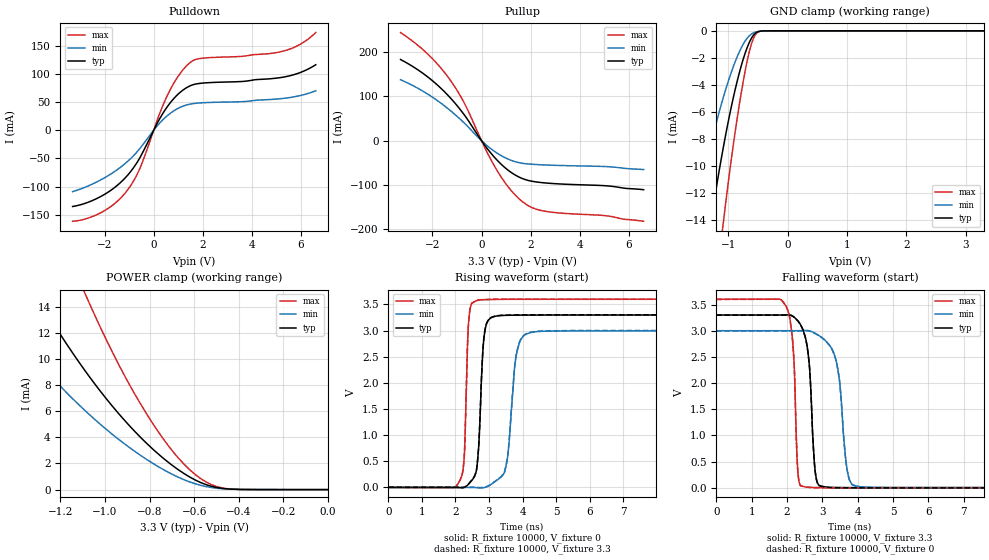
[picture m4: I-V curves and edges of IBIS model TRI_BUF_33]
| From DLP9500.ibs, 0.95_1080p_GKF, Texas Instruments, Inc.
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[Model]   TRI_BUF_33
Model_type  3-state
Enable   Active-High
Vref =   0
Rref =   10000
Cref =   0p
Vmeas =   1.5
| variable   typ   min   max
C_comp   1.64pF   1.51pF   2.01pF
| C_pullup   3.64pF   2.66pF   4.74pF
| C_pulldown   2.77pF   1.94pF   3.37pF
| C_tri-state   1.64pF   1.51pF   2.01pF
[Temperature Range]   40   125   -40
| Ambient temperature   25   110   -40
[Voltage range]   3.3   3   3.6
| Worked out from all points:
|   slope of the pulldown table from 0 to 0.495 V, typ, clamps not added: 12.9 ohm
|   slope of the pullup table from 0 to 0.495 V, typ, clamps not added: 13.9 ohm
|   GND clamp passes 1 mA (typ) near -0.66 V on its own axis
|   POWER clamp passes 1 mA (typ) near -0.62 V on its own axis
|   rising waveform, R_fixture 10000, V_fixture 0: 20-80 % time 141ps typ, 224ps min, 96.6ps max; typ from 0 V to 3.3 V
|   falling waveform, R_fixture 10000, V_fixture 3.3: 20-80 % time 174ps typ, 253ps min, 128ps max; typ from 3.3 V to 0.004 V
|   rising waveform, R_fixture 10000, V_fixture 3.3: 20-80 % time 141ps typ, 224ps min, 96.6ps max; typ from 0.004 V to 3.3 V
|   falling waveform, R_fixture 10000, V_fixture 0: 20-80 % time 174ps typ, 253ps min, 127ps max; typ from 3.3 V to 0 V
[GND Clamp]
| TRI_BUF_33
|   Voltage   I(typ)   I(min)   I(max)
-3.3V     -90.74mA   -64.34mA   -120.4mA
-1.58V    -23.02mA   -14.24mA   -35.11mA
-1.315V   -14.82mA   -8.851mA   -23.44mA
-1.28V    -13.82mA   -8.21mA    -21.98mA
-1.08V    -8.591mA   -4.902mA   -14.14mA
-935mV    -5.377mA   -2.918mA   -9.123mA
-795mV    -2.828mA   -1.398mA   -4.995mA
-670mV    -1.125mA   -492uA     -2.021mA
-575mV    -328.8uA   -155.1uA   -571.2uA
-500mV    -70.88uA   -51.22uA   -102.5uA
-375mV    -2.475uA   -4.552uA   -1.459uA
3.3V      49.59pA    1.106uA    33.03pA
[POWER Clamp]
| TRI_BUF_33
|   Voltage   I(typ)   I(min)   I(max)
-3.3V     108mA      77.88mA    156.4mA
-1.545V   22.36mA    15.03mA    36.12mA
-1.3V     14.64mA    9.77mA     23.97mA
-1.095V   9.233mA    6.138mA    15.22mA
-1.075V   8.762mA    5.822mA    14.45mA
-945mV    5.943mA    3.931mA    9.788mA
-805mV    3.41mA     2.22mA     5.575mA
-705mV    1.945mA    1.23mA     3.121mA
-595mV    732.7uA    446uA      1.151mA
-525mV    266uA      165.6uA    400.3uA
-440mV    41.44uA    31.47uA    49.29uA
-48.03fV  49.59pA    201.8pA    43.32pA
[Pulldown]
| TRI_BUF_33
|   Voltage   I(typ)   I(min)   I(max)
-3.3V     -135.4mA   -109mA     -161.7mA
-2.03V    -114.7mA   -85.13mA   -143.6mA
-1.045V   -78.98mA   -54.56mA   -105mA
-555mV    -48.27mA   -31.88mA   -67.09mA
220mV     18.6mA     11.64mA    27.17mA
600mV     44.67mA    27.61mA    65.86mA
1.045V    66.29mA    40.16mA    99.13mA
1.5V      79.42mA    46.79mA    121mA
1.97V     83.91mA    48.95mA    128.2mA
5.21V     94.09mA    56.42mA    140.1mA
5.945V    102.4mA    61.6mA     152.4mA
6.6V      116.6mA    70.3mA     173.8mA
[Pullup]
| TRI_BUF_33
|   Voltage   I(typ)   I(min)   I(max)
-3.3V     183.6mA    137.8mA    244.4mA
-2.205V   144.7mA    105.8mA    196.6mA
-1.31V    99.19mA    69.94mA    139.7mA
-695mV    57.8mA     39.52mA    84.19mA
140mV     -10.9mA    -7.086mA   -16.47mA
615mV     -42.85mA   -27.33mA   -65.74mA
1.15V     -69.42mA   -43.04mA   -108.8mA
1.68V     -85.76mA   -51.11mA   -138.3mA
2.105V    -91.99mA   -53.34mA   -152.2mA
2.63V     -95.51mA   -54.82mA   -159.7mA
5.005V    -101.5mA   -58.24mA   -169.1mA
6.6V      -110.6mA   -65.14mA   -182mA
[Ramp]
| TRI_BUF_33
| variable   typ   min   max
dV/dt_r   1.98/1.49E-10   1.80/2.36E-10   2.16/1.03E-10
dV/dt_f   1.98/1.77E-10   1.80/2.56E-10   2.16/1.29E-10
R_load = 10000
[Rising Waveform]
| TRI_BUF_33
R_fixture =   10000
C_fixture =   0
L_fixture =   0
V_fixture =   0
V_fixture_min = 0
V_fixture_max = 0
|   Time   V(typ)   V(min)   V(max)
0s        920.7pV    4.06nV     601pV
2.14ns    -4.487mV   139.3uV    142.8mV
2.265ns   1.174mV    246.3uV    626.8mV
2.4ns     71.01mV    -37.67uV   3.22V
2.665ns   557.9mV    -4.992mV   3.577V
2.93ns    3.137V     11.71mV    3.591V
3.47ns    3.289V     311.6mV    3.596V
3.815ns   3.293V     2.54V      3.597V
4.225ns   3.295V     2.959V     3.597V
23ns      3.296V     2.994V     3.597V
[Falling Waveform]
| TRI_BUF_33
R_fixture =   10000
C_fixture =   0
L_fixture =   0
V_fixture =   3.3
V_fixture_min = 3
V_fixture_max = 3.6
|   Time   V(typ)   V(min)   V(max)
0s        3.3V       3V         3.6V
1.985ns   3.302V     3V         3.457V
2.18ns    3.271V     3V         2.632V
2.32ns    3.18V      3V         232.1mV
2.5ns     2.923V     3.004V     19.74mV
2.8ns     313.1mV    2.951V     6.608mV
2.98ns    31.35mV    2.876V     4.673mV
3.395ns   6.65mV     2.423V     3.14mV
3.95ns    4.082mV    37.68mV    2.783mV
23ns      3.639mV    5.256mV    2.73mV
[Rising Waveform]
| TRI_BUF_33
R_fixture =   10000
C_fixture =   0
L_fixture =   0
V_fixture =   3.3
V_fixture_min = 3
V_fixture_max = 3.6
|   Time   V(typ)   V(min)   V(max)
0s        3.639mV    5.256mV    2.73mV
2.14ns    -827.2uV   5.394mV    146.2mV
2.265ns   4.91mV     5.498mV    634mV
2.4ns     75.12mV    5.212mV    3.226V
2.665ns   569mV      298.7uV    3.58V
2.93ns    3.143V     17.28mV    3.594V
3.47ns    3.293V     324.1mV    3.599V
3.815ns   3.297V     2.556V     3.6V
4.225ns   3.299V     2.966V     3.6V
23ns      3.3V       3V         3.6V
[Falling Waveform]
| TRI_BUF_33
R_fixture =   10000
C_fixture =   0
L_fixture =   0
V_fixture =   0
V_fixture_min = 0
V_fixture_max = 0
|   Time   V(typ)   V(min)   V(max)
0s        3.296V     2.994V     3.597V
1.985ns   3.298V     2.994V     3.454V
2.18ns    3.267V     2.994V     2.626V
2.32ns    3.176V     2.995V     227.6mV
2.5ns     2.917V     2.998V     16.86mV
2.795ns   335.9mV    2.947V     3.923mV
2.98ns    27.42mV    2.869V     1.925mV
3.395ns   2.962mV    2.413V     406.4uV
3.95ns    435.7uV    31.71mV    52.61uV
23ns      -7.923nV   13.92nV    -5.083nV
